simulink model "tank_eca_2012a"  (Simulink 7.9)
settings: Solver=ode3  StartTime=0.0  StopTime=simopt.Tf  FixedStep=simopt.h  RelTol=1e-3
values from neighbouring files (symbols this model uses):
  simopt = []    [setParams.m]
libraries: cstblocks x2

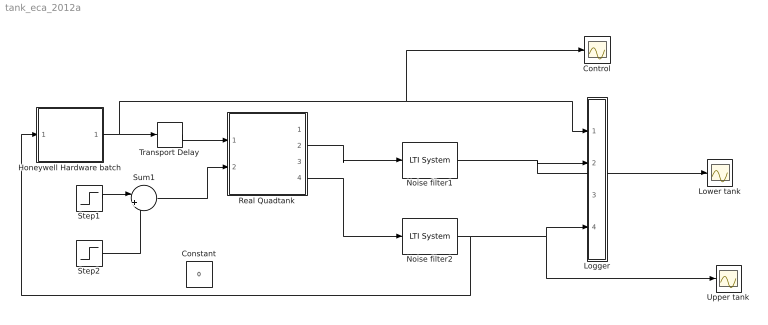
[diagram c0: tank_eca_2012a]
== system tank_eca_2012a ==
  Constant : Constant  Value=0
  Control : Scope
  Honeywell Hardware batch : Subsystem
  Logger : Subsystem
  Lower tank : Scope
  Noise filter1 : cstblocks/LTI System  sys=simopt.F  IC=[]
  Noise filter2 : cstblocks/LTI System  sys=simopt.F  IC=[]
  Real Quadtank : Subsystem  AncestorBlock=tank/Real Quadtank  mask{h=0.01}
  Step1 : Step  Time=300  Before=2  After=3  SampleTime=simopt.h
  Step2 : Step  Time=1000  SampleTime=simopt.h
  Sum1 : Sum  Inputs=|+-
  Transport Delay : TransportDelay  DelayTime=20
  Upper tank : Scope
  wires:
  Noise filter1/1 -> Lower tank/1, Logger/2(y1)
  Noise filter2/1 -> Logger/4(y2), Upper tank/1, Honeywell Hardware batch/1("[ y ]")
  Real Quadtank/2(y2) -> Noise filter1/1
  Real Quadtank/4(y4) -> Noise filter2/1
  Honeywell Hardware batch/1("[  u ]") -> Logger/1(u1), Control/1, Transport Delay/1
  Transport Delay/1 -> Real Quadtank/1(u1)
  Step1/1 -> Sum1/1
  Step2/1 -> Sum1/2
  Sum1/1 -> Real Quadtank/2(u2)

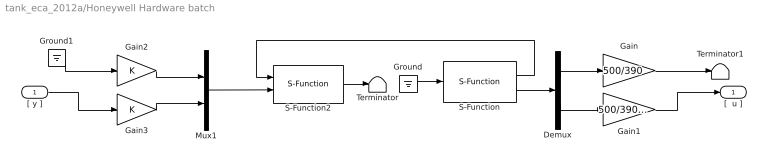
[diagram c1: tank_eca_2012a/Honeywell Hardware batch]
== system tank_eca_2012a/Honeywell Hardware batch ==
  "[ y ]" : Inport
  Demux : Demux  Outputs=2
  Gain : Gain  Gain=500/390
  Gain1 : Gain  Gain=500/390*10/9.35
  Gain2 : Gain
  Gain3 : Gain
  Ground : Ground
  Ground1 : Ground
  Mux1 : Mux  Inputs=2
  S-Function : S-Function  FunctionName=analogin  Parameters=simopt.h [1 0]  EnableBusSupport=off
  S-Function2 : S-Function  FunctionName=analogout  Parameters=simopt.h [1 0]  EnableBusSupport=off
  Terminator : Terminator
  Terminator1 : Terminator
  "[  u ]" : Outport  InitialOutput=0
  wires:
  Gain3/1 -> Mux1/2
  Gain2/1 -> Mux1/1
  Gain1/1 -> "[  u ]"/1
  Demux/2 -> Gain1/1
  Demux/1 -> Gain/1
  Gain/1 -> Terminator1/1
  Ground1/1 -> Gain2/1
  "[ y ]"/1 -> Gain3/1
  Mux1/1 -> S-Function2/2
  S-Function/2 -> Demux/1
  S-Function/1 -> S-Function2/1
  S-Function2/1 -> Terminator/1
  Ground/1 -> S-Function/1

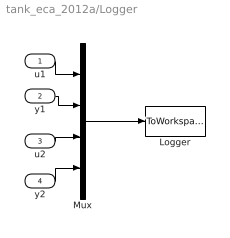
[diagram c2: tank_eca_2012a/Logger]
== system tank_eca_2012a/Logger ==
  u1 : Inport  SampleTime=simopt.h
  y1 : Inport  Port=2  SampleTime=simopt.h
  u2 : Inport  Port=3  SampleTime=simopt.h
  y2 : Inport  Port=4  SampleTime=simopt.h
  Logger : ToWorkspace  VariableName=simout  SampleTime=simopt.h  SaveFormat=Structure With Time
  Mux : Mux
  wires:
  Mux/1 -> Logger/1
  u1/1 -> Mux/1
  y1/1 -> Mux/2
  u2/1 -> Mux/3
  y2/1 -> Mux/4

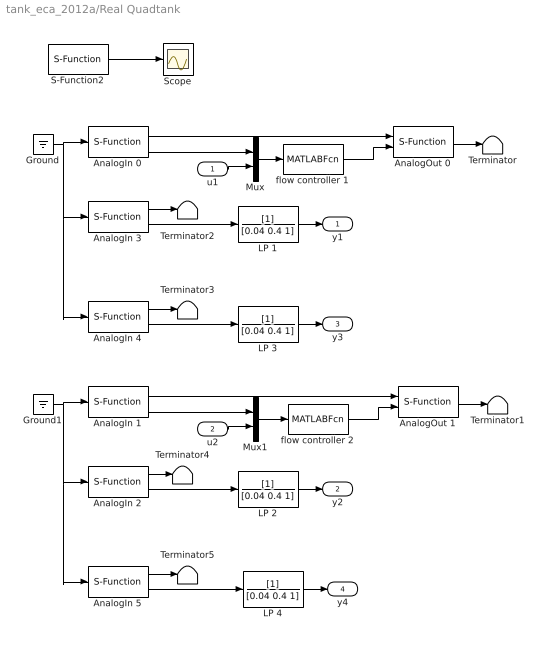
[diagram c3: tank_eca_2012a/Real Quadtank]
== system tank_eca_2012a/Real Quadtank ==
  u1 : Inport
  u2 : Inport  Port=2
  AnalogIn 0 : S-Function  FunctionName=analogin  Parameters=h [35]  EnableBusSupport=off
  AnalogIn 1 : S-Function  FunctionName=analogin  Parameters=h [34]  EnableBusSupport=off
  AnalogIn 2 : S-Function  FunctionName=analogin  Parameters=h [33]  EnableBusSupport=off
  AnalogIn 3 : S-Function  FunctionName=analogin  Parameters=h [31]  EnableBusSupport=off
  AnalogIn 4 : S-Function  FunctionName=analogin  Parameters=h [30]  EnableBusSupport=off
  AnalogIn 5 : S-Function  FunctionName=analogin  Parameters=h [32]  EnableBusSupport=off
  AnalogOut 0 : S-Function  FunctionName=analogout  Parameters=h [31]  EnableBusSupport=off
  AnalogOut 1 : S-Function  FunctionName=analogout  Parameters=h [30]  EnableBusSupport=off
  Ground : Ground
  Ground1 : Ground
  LP {1..4} (4 alike) : TransferFcn  Denominator=[0.04 0.4 1]
  Mux : Mux  Inputs=2
  Mux1 : Mux  Inputs=2
  S-Function2 : S-Function  FunctionName=realtimer  Parameters=h  EnableBusSupport=off
  Scope : Scope
  Terminator{,1..5} (6 alike) : Terminator
  flow controller 1 : MATLABFcn  MATLABFcn=flowCtrl1  SampleTime=0.01
  flow controller 2 : MATLABFcn  MATLABFcn=flowCtrl2  SampleTime=0.01
  y1 : Outport
  y2 : Outport  Port=2
  y3 : Outport  Port=3
  y4 : Outport  Port=4
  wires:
  LP 4/1 -> y4/1
  LP 2/1 -> y2/1
  LP 3/1 -> y3/1
  LP 1/1 -> y1/1
  AnalogIn 0/2 -> Mux/1
  AnalogIn 1/2 -> Mux1/1
  flow controller 2/1 -> AnalogOut 1/2
  Mux1/1 -> flow controller 2/1
  u2/1 -> Mux1/2
  flow controller 1/1 -> AnalogOut 0/2
  Mux/1 -> flow controller 1/1
  u1/1 -> Mux/2
  AnalogIn 5/1 -> Terminator5/1
  AnalogIn 2/1 -> Terminator4/1
  Ground1/1 -> AnalogIn 1/1, AnalogIn 2/1, AnalogIn 5/1
  AnalogIn 5/2 -> LP 4/1
  AnalogIn 2/2 -> LP 2/1
  AnalogIn 4/1 -> Terminator3/1
  AnalogIn 3/1 -> Terminator2/1
  Ground/1 -> AnalogIn 4/1, AnalogIn 3/1, AnalogIn 0/1
  AnalogIn 4/2 -> LP 3/1
  AnalogIn 3/2 -> LP 1/1
  AnalogOut 1/1 -> Terminator1/1
  AnalogIn 1/1 -> AnalogOut 1/1
  AnalogOut 0/1 -> Terminator/1
  AnalogIn 0/1 -> AnalogOut 0/1
  S-Function2/1 -> Scope/1
